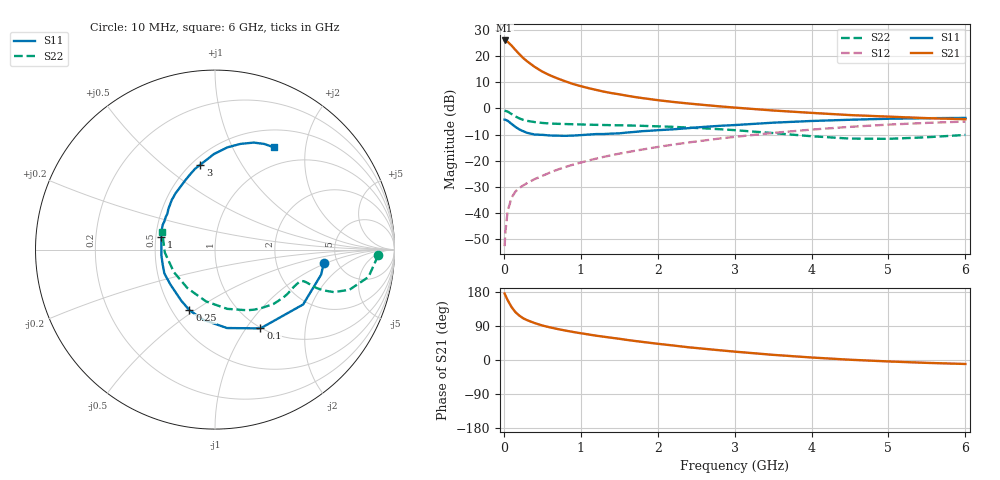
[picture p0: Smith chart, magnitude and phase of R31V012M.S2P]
! SIEMENS Small Signal Semiconductors
! BFR181
! Si NPN RF Bipolar Junction Transistor in SOT23
! VCE = 1 V  IC = 12 mA
! Common Emitter S-Parameters:  May  1996
# GHz  S  MA  R  50
!  f  S11  S21  S12  S22
! GHz  MAG  ANG  MAG  ANG  MAG  ANG  MAG  ANG
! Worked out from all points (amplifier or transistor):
!   36 points, 10 MHz to 6 GHz, reference 50 ohm
!   highest |S21| = 26.0 dB at 10 MHz (marker M1)
!   |S21| within 3 dB of that: start of sweep to 131.7 MHz
!   unconditionally stable (mu >= 1): start of sweep to 13.49 MHz; 295.4 MHz to end of sweep
!   at 250 MHz: K = 0.92, MSG = 24.4 dB, |S12| = -29.6 dB
!   at 1.4 GHz: K = 1.35, MAG = 8.4 dB, |S12| = -17.9 dB
!   at 6 GHz: K = 1.07, MAG = -1.2 dB, |S12| = -5.0 dB
!   S11 on the Smith chart (normalised r, x): 10 MHz: 3.90, -0.91; 100 MHz: 0.99, -1.17; 250 MHz: 0.61, -0.48; 1 GHz: 0.53, +0.09; 3 GHz: 0.55, +0.68; 6 GHz: 0.73, +1.47
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0.01  0.6103 -6.9  20.01 175.3  0.0023 82.3  0.9084 -2.0
0.02  0.6077 -13.2  19.72 170.6  0.0043 85.6  0.896 -4.3
0.05  0.5784 -31.9  18.84 157.8  0.0109 76.7  0.8689 -10.1
0.1  0.5068 -60.0  15.99 139.8  0.0194 66.6  0.7809 -16.7
0.15  0.4421 -81.3  13.21 126.5  0.0255 61.6  0.7025 -19.7
0.2  0.3969 -99.1  10.99 117.3  0.0298 61.0  0.6454 -20.6
0.25  0.3667 -112.8  9.267 110.3  0.0333 60.4  0.6047 -20.7
0.3  0.3412 -123.4  8.037 105.3  0.037 62.1  0.5779 -20.4
0.4  0.3159 -141.5  6.25 97.5  0.0442 62.8  0.5473 -19.8
0.5  0.3118 -154.8  5.064 91.1  0.0511 64.8  0.5266 -19.6
0.6  0.3028 -164.6  4.296 86.1  0.0591 66.1  0.5141 -19.9
0.7  0.3003 -173.6  3.741 81.7  0.0674 67.2  0.5066 -20.5
0.9  0.3014 172.0  2.937 74.0  0.0837 68.3  0.4975 -22.2
1  0.3078 166.3  2.667 70.6  0.0918 68.9  0.4928 -23.3
1.1  0.3154 160.1  2.446 67.4  0.1006 69.0  0.4882 -24.6
1.6  0.345 138.8  1.75 53.0  0.1447 67.9  0.4721 -31.9
2.2  0.3977 119.3  1.33 38.3  0.2023 64.1  0.4441 -43.1
3  0.4796 99.9  1.037 22.1  0.2848 56.5  0.3832 -61.9
3.5  0.5327 90.6  0.912 13.6  0.3393 50.7  0.337 -78.4
4.5  0.6065 76.3  0.745 0.7  0.4437 36.9  0.2642 -125.5
5.5  0.6495 65.0  0.651 -7.6  0.528 22.2  0.2801 -176.7
6  0.6575 60.1  0.621 -10.5  0.5602 14.6  0.3108 161.3
